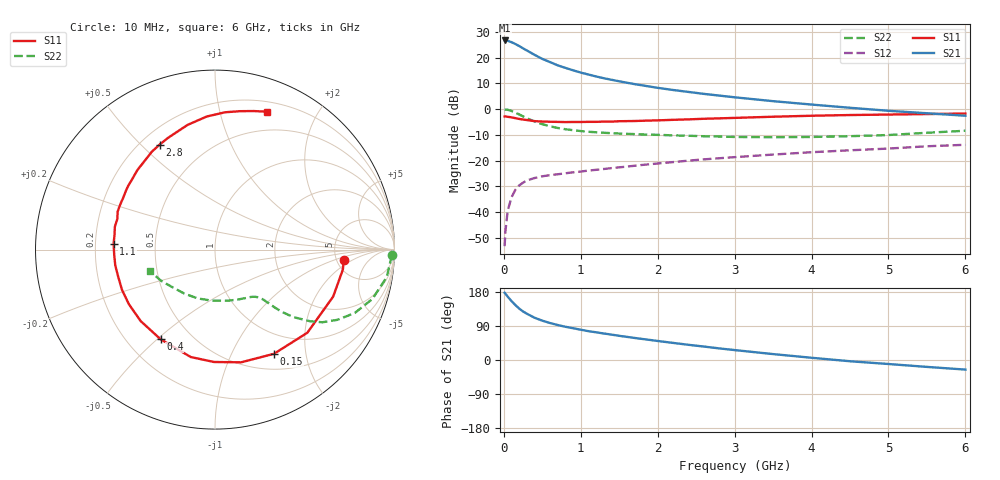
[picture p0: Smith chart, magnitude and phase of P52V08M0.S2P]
! SIEMENS Small Signal Semiconductors
! BFP183
! Si NPN RF Bipolar Junction Transistor in SOT143
! VCE = 2 V  IC = 8 mA
! Common Emitter S-Parameters:  March  1996
# GHz  S  MA  R  50
!  f  S11  S21  S12  S22
! GHz  MAG  ANG  MAG  ANG  MAG  ANG  MAG  ANG
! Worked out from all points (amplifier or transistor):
!   36 points, 10 MHz to 6 GHz, reference 50 ohm
!   highest |S21| = 26.6 dB at 10 MHz (marker M1)
!   |S21| within 3 dB of that: start of sweep to 246.4 MHz
!   unconditionally stable (mu >= 1): 1.238 GHz to 5.655 GHz
!   at 250 MHz: K = 0.29, MSG = 26.0 dB, |S12| = -28.5 dB
!   at 1.4 GHz: K = 1.06, MAG = 15.6 dB, |S12| = -22.9 dB
!   at 6 GHz: K = 0.96, MSG = 5.6 dB, |S12| = -13.8 dB
!   lowest NFmin = 1.30 dB at 450 MHz
!   S11 on the Smith chart (normalised r, x): 10 MHz: 5.81, -1.36; 150 MHz: 0.70, -1.47; 400 MHz: 0.34, -0.51; 1.1 GHz: 0.28, +0.03; 2.8 GHz: 0.27, +0.57; 6 GHz: 0.30, +1.40
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0.01  0.7198 -4.5  21.42 177.5  0.0022 83.8  0.9871 -1.8
0.02  0.7211 -8.9  21.4 175.2  0.0042 88.5  0.9799 -3.7
0.05  0.7085 -21.7  21.08 167.2  0.0107 82.2  0.969 -9.1
0.1  0.6923 -42.0  19.81 155.4  0.0195 69.3  0.9191 -17.4
0.15  0.667 -60.5  18.26 144.8  0.0273 62.1  0.855 -24.4
0.2  0.6446 -77.0  16.69 135.7  0.0332 56.5  0.7869 -29.8
0.25  0.6262 -90.5  15.05 128.0  0.0375 51.5  0.7222 -34.1
0.3  0.6136 -102.7  13.67 122.0  0.0414 47.8  0.6634 -37.0
0.4  0.5842 -121.3  11.25 111.5  0.0461 42.7  0.5749 -40.8
0.5  0.5745 -136.1  9.411 103.8  0.0498 39.6  0.5102 -42.9
0.6  0.5681 -147.5  8.152 97.6  0.0524 38.7  0.4638 -44.1
0.7  0.5647 -156.5  7.058 92.3  0.0545 37.6  0.4306 -44.8
0.8  0.5601 -164.6  6.295 87.7  0.0569 37.8  0.4069 -45.4
1.1  0.5659 176.6  4.681 76.1  0.0643 38.2  0.3635 -47.4
1.3  0.5724 167.1  3.964 69.9  0.069 38.5  0.3474 -49.3
1.6  0.5848 154.6  3.245 61.0  0.0768 39.3  0.3312 -52.8
2.2  0.6192 134.3  2.347 45.1  0.0939 39.2  0.3096 -62.9
2.8  0.6613 117.8  1.827 30.6  0.1114 37.1  0.2937 -76.0
3.5  0.7114 102.4  1.425 15.6  0.1314 33.6  0.2849 -94.2
4.5  0.7671 85.8  1.061 -3.3  0.159 27.0  0.2984 -124.3
5.5  0.8011 74.5  0.831 -18.2  0.1902 20.6  0.3473 -150.0
6  0.8209 69.4  0.743 -25.3  0.2033 16.3  0.3806 -161.6
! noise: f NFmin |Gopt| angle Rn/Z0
0.45  1.3  0.17  43  0.21
0.9  1.35  0.21  115  0.2
1.8  2.05  0.33  -177  0.14
